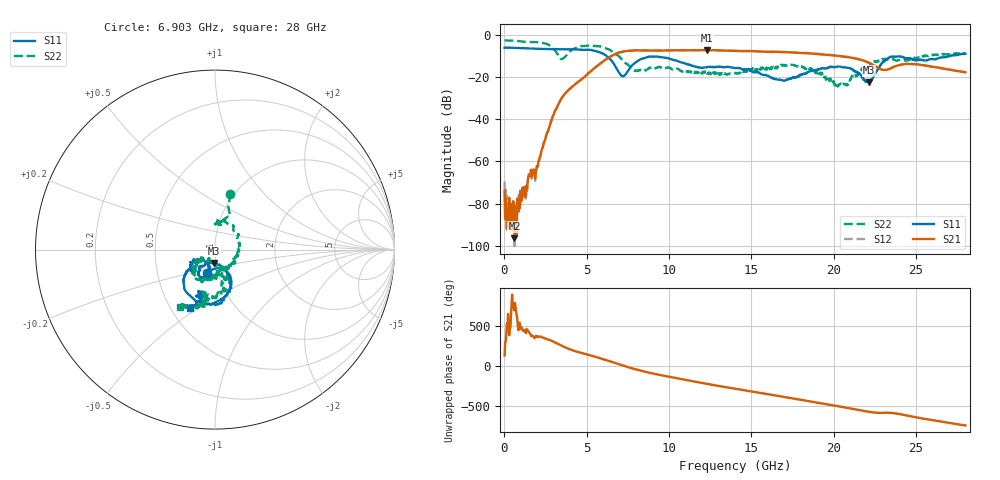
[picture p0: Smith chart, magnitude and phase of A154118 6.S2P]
!  2-Port S-parameters saved by WinCal
! VAR MeasName=S-Parameters (CALIBRATED_DATA) read from VNA (N5230A)
! VAR MeasDate=2015-9-10 14:34:53
! VAR NAME=A154118 6
! VAR FILENAME=A154118 6.S2P
! VAR DATE=2015-9-10 14:34:53
! VAR PHYS_PORTS=1,2
# Hz S DB R 50
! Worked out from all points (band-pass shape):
!   801 points, 10 MHz to 28 GHz, reference 50 ohm
!   highest |S21| = -7.20 dB at 12.29 GHz (marker M1); lowest = -96.4 dB at 604.8 MHz (marker M2)
!   |S21| within 3 dB of the highest: 6.469 GHz to 20.49 GHz (14.02 GHz wide, 104 % of centre)
!   lowest |S11| = -22.6 dB at 22.12 GHz (marker M3), VSWR 1.16, Z = 48.9 - j7.29 ohm
!   |S11| at or under -10 dB: 6.194 GHz to 27.06 GHz (20.86 GHz wide, 125 % of centre)
!   |S22| runs from -25.0 to -2.7 dB; largest |S21 - S12| = 0.0087
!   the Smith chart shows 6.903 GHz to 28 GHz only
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1e7  -6.09 179.6  -73.96 133.7  -69.47 -47.5  -2.67 179.8
1.849375e8  -6.06 173.7  -82.45 123.8  -78.90 74.3  -2.69 175.4
6.047875e8  -6.19 159.8  -96.43 -18.4  -100.13 -148.1  -2.80 165.2
1.934312e9  -6.61 116.6  -64.10 21.1  -64.35 21.3  -3.44 130.6
2.494112e9  -6.69 96.0  -48.85 -12.7  -48.89 -12.4  -4.13 102.5
3.193862e9  -6.78 67.7  -34.34 -74.0  -34.32 -73.7  -8.71 25.6
3.753662e9  -6.85 42.4  -27.19 -130.2  -27.18 -129.9  -9.84 -109.0
4.698325e9  -7.08 -5.3  -20.99 163.5  -20.98 163.6  -5.38 165.9
5.817925e9  -8.40 -67.5  -13.69 99.6  -13.61 99.9  -5.48 117.6
7.182438e9  -19.57 -82.5  -7.98 7.3  -7.91 7.2  -12.27 71.7
8.232062e9  -11.74 -75.1  -7.41 -55.4  -7.32 -55.7  -16.61 86.9
9.351662e9  -10.40 -112.6  -7.50 -107.3  -7.39 -107.7  -15.29 73.7
1.082114e10  -13.15 -139.9  -7.33 -166.6  -7.25 -167.4  -17.44 19.1
1.229061e10  -15.31 -137.5  -7.20 137.5  -7.18 136.9  -17.55 -37.2
1.4005e10  -15.70 -146.3  -7.63 75.7  -7.61 75.0  -18.24 -81.8
1.634916e10  -20.85 -143.7  -8.06 -4.9  -8.08 -5.3  -15.91 -104.2
1.869332e10  -16.89 -104.5  -8.88 -87.8  -8.86 -88.0  -16.24 -136.9
2.019779e10  -15.12 -117.3  -9.92 -141.8  -9.86 -142.6  -23.95 -126.9
2.21221e10  -22.58 -94.2  -13.20 145.8  -13.15 145.1  -14.94 -70.8
2.334666e10  -10.85 -80.3  -16.24 133.6  -16.18 132.9  -11.78 -95.9
2.488611e10  -11.89 -108.4  -13.85 81.1  -13.89 80.2  -10.81 -98.6
2.8e10  -8.98 -113.3  -17.74 -26.3  -17.76 -27.4  -8.52 -120.8
